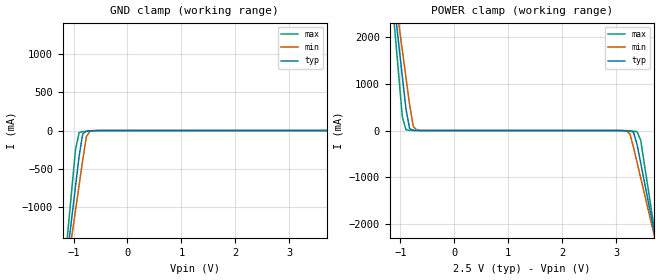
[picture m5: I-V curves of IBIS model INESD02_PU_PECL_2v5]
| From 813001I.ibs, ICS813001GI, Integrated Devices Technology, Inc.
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[Model] INESD02_PU_PECL_2v5
Model_type   Input
Polarity   Non-Inverting
Vinl = 1.4V
Vinh = 1.85V
|   typ   min   max
C_comp   2pF   1.5pF   2.5pF
|   typ   min   max
[Voltage range]  2.5V   2.375V   2.625V
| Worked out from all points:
|   GND clamp passes 1 mA (typ) near -0.59 V on its own axis
|   POWER clamp passes 1 mA (typ) near -0.70 V on its own axis
[GND_clamp]
|Voltage   I(typ)   I(min)   I(max)
-3.3V     -3.894A    -3.674A    -4.294A
-1.098V   -1.521A    -1.7A      -1.261A
-963.9mV  -730.3mA   -1.043A    -249.9mA
-829.9mV  -43.34mA   -386.7mA   -14.26mA
-628.9mV  -1.599mA   -1.763mA   -3.5mA
3.995V    711.6uA    10.32mA    481.3uA
4.062V    4.029mA    88.04mA    1.401mA
4.196V    445.8mA    1.124A     14.79mA
4.263V    1.139A     1.7A       275.9mA
4.33V     1.832A     2.277A     1.163A
4.397V    2.525A     2.854A     2.05A
6.6V      8.773A     8.051A     10.04A
[POWER_clamp]
|Voltage   I(typ)   I(min)   I(max)
-3.3V     6.7A       6.327A     7.39A
-1.165V   3.23A      3.44A      2.951A
-1.098V   2.536A     2.863A     2.063A
-1.031V   1.842A     2.286A     1.176A
-963.9mV  1.149A     1.709A     289.6mA
-896.9mV  456.4mA    1.132A     15.33mA
-762.9mV  4.159mA    91.01mA    1.421mA
-695.9mV  727.9uA    10.67mA    490.4uA
3.191V    -3.204mA   -9.193mA   -6.2mA
3.392V    -305mA     -689.5mA   -24.7mA
3.727V    -2.281A    -2.333A    -2.233A
6.6V      -9.799A    -8.591A    -11.84A
